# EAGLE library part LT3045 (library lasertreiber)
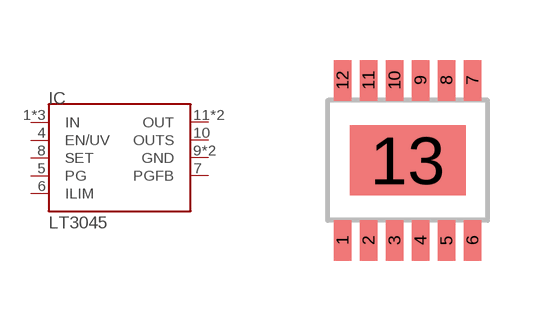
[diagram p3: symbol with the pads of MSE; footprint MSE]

Designator prefix IC

## LT3045  [MSE]
1  IN  in
2  IN  in
3  IN  in
4  EN/UV
5  PG
6  ILIM
7  PGFB
8  SET
9  GND
10  OUTS  out
11  OUT  out
12  OUT  out
13  GND

## Footprint MSE (pad centres in mm)
smd 0.445 x 1.016: 1 -1.626,-2; 2 -0.975,-2; 3 -0.325,-2; 4 0.325,-2; 5 0.975,-2; 6 1.626,-2; 7 1.626,2; 8 0.975,2; 9 0.325,2; 10 -0.325,2; 11 -0.975,2; 12 -1.626,2
smd 2.9 x 1.75: 13 0,0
